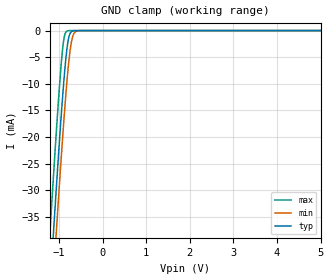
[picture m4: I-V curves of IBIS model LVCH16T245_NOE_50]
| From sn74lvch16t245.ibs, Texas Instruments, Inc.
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[Model]   LVCH16T245_NOE_50
Model_type  Input
Vinl=1.35
Vinh=3.85
| variable   typ   min   max
C_comp   2.83pF   2.20pF   4.18pF
[Temperature Range]   40   100   -40
| Ambient temperature   25   85   -40
[Voltage range]   5   4.5   5.5
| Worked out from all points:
|   GND clamp passes 1 mA (typ) near -0.77 V on its own axis
[GND Clamp]
| LVCH16T245_NOE_50
|   Voltage   I(typ)   I(min)   I(max)
-5.5V     -655.2mA   -662.2mA   -646.6mA
-1.215V   -49.6mA    -57.88mA   -38.96mA
-1.135V   -39.07mA   -47.36mA   -28.42mA
-1.115V   -36.48mA   -44.76mA   -25.84mA
-1.055V   -28.82mA   -37.05mA   -18.27mA
-915mV    -12.21mA   -19.95mA   -3.333mA
-870mV    -7.651mA   -14.9mA    -891.1uA
-815mV    -3.252mA   -9.299mA   -87.06uA
-770mV    -1.128mA   -5.445mA   -10.73uA
-705mV    -146.7uA   -1.723mA   -505nA
-575mV    -1.597uA   -52.97uA   -1.117nA
5V        9.69pA     12.83pA    9.218pA
